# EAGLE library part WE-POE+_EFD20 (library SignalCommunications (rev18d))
WE-PoE+ Power over Ethernet Plus Transformer Characteristics Designed to meet 25 W PoE+ requirements of IEEE802.3at Frequency range: 250–400 kHz Input voltage range: 36–72 V 1.5 kV Hipot test between primary and secondary Operating temperature: –40 °C to +125 °C Applications PoE+ powered devices IP phones WLAN-Access points Security cameras Details see: http://katalog.we-online.de/en/pbs/WE-POE-PLUS?m Updated by Dan Xu 2014-07-08 2014 (C) Wurth Elektronik
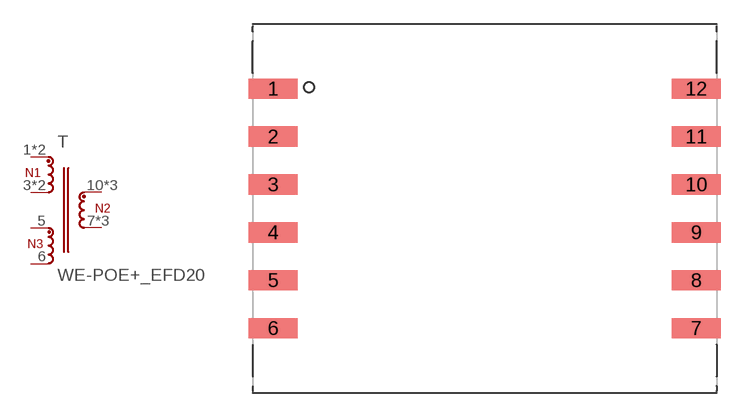
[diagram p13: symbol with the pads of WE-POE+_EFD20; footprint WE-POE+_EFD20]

Designator prefix T

## WE-POE+_EFD20_749119433, WE-POE+_EFD20_7491194501, WE-POE+_EFD20_7491194912  [WE-POE+_EFD20]
1  1  pas
2  1  pas
3  6  pas
4  6  pas
5  5  pas
6  4  pas
7  3  pas
8  3  pas
9  3  pas
10  2  pas
11  2  pas
12  2  pas

## Footprint WE-POE+_EFD20 (pad centres in mm)
Transformer, EFD20 SMD 12 Pin
smd 3.05 x 1.27: 1 -13.26,7.5; 2 -13.26,4.5; 3 -13.26,1.5; 4 -13.26,-1.5; 5 -13.26,-4.5; 6 -13.26,-7.5; 7 13.26,-7.5; 8 13.26,-4.5; 9 13.26,-1.5; 10 13.26,1.5; 11 13.26,4.5; 12 13.26,7.5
